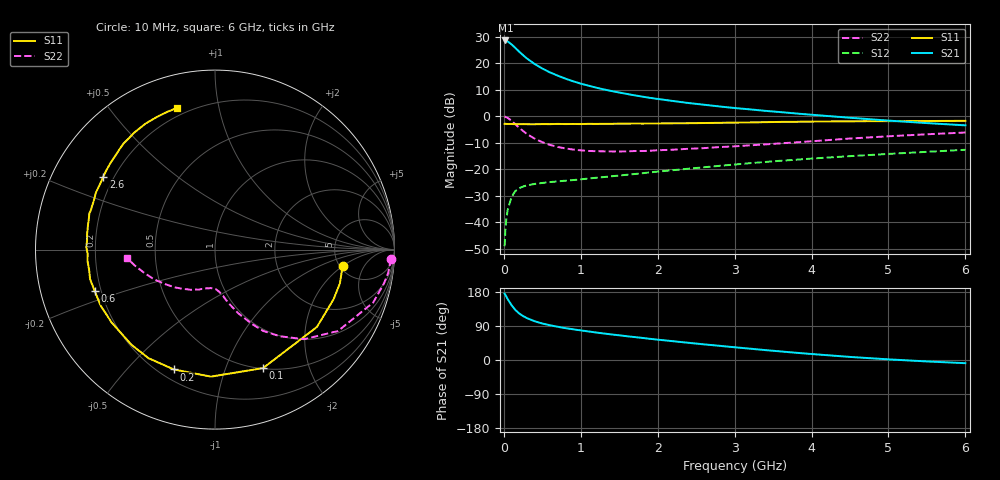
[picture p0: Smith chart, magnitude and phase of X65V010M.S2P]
! SIEMENS Small Signal Semiconductors
! BFP193W
! Si NPN RF Bipolar Junction Transistor in SOT343
! VCE = 5 V  IC = 10 mA
! Common Emitter S-Parameters:  April 1994
# GHz  S  MA  R  50
!  f  S11  S21  S12  S22
! GHz  MAG  ANG  MAG  ANG  MAG  ANG  MAG  ANG
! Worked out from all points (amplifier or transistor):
!   40 points, 10 MHz to 6 GHz, reference 50 ohm
!   highest |S21| = 28.6 dB at 20 MHz (marker M1)
!   |S21| within 3 dB of that: start of sweep to 156.1 MHz
!   unconditionally stable (mu >= 1): 1.325 GHz to 4.237 GHz
!   at 200 MHz: K = 0.22, MSG = 25.8 dB, |S12| = -27.2 dB
!   at 1.5 GHz: K = 1.05, MAG = 14.3 dB, |S12| = -22.4 dB
!   at 6 GHz: K = 0.92, MSG = 4.6 dB, |S12| = -12.7 dB
!   lowest NFmin = 1.30 dB at 450 MHz
!   S11 on the Smith chart (normalised r, x): 10 MHz: 5.28, -2.01; 100 MHz: 0.51, -1.36; 200 MHz: 0.26, -0.68; 600 MHz: 0.18, -0.16; 2.6 GHz: 0.16, +0.29; 6 GHz: 0.16, +0.76
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0.01  0.7169 -7.4  26.98 175.1  0.0035 87.1  0.9816 -3.0
0.02  0.7209 -15.2  27.01 172.0  0.0071 80.8  0.9734 -7.7
0.03  0.7163 -22.7  26.71 168.2  0.0105 80.2  0.9599 -11.4
0.05  0.7129 -37.2  25.87 160.7  0.017 73.1  0.9294 -18.5
0.1  0.7123 -67.9  22.78 144.7  0.0296 59.7  0.822 -33.5
0.15  0.7081 -91.8  19.51 131.9  0.0386 49.7  0.7036 -45.2
0.2  0.706 -108.9  16.54 122.7  0.0435 43.3  0.6029 -53.2
0.25  0.7095 -121.5  14.24 115.9  0.047 38.8  0.5264 -59.4
0.3  0.7055 -131.3  12.34 110.5  0.0492 35.7  0.4607 -63.7
0.4  0.7048 -144.8  9.714 102.3  0.0525 32.6  0.3769 -70.0
0.5  0.7098 -154.0  7.97 96.3  0.0548 31.6  0.3229 -74.3
0.6  0.7088 -161.0  6.728 91.6  0.0569 31.4  0.2869 -77.7
0.8  0.7102 -171.1  5.13 84.1  0.0605 32.8  0.2464 -82.5
1.1  0.7173 178.8  3.781 75.3  0.0665 35.8  0.2206 -88.6
1.3  0.718 173.1  3.207 69.9  0.0708 37.9  0.2167 -92.4
1.6  0.7234 166.3  2.632 62.7  0.0782 40.9  0.2169 -97.7
2.2  0.7357 154.3  1.938 49.6  0.0955 44.5  0.2329 -109.2
2.6  0.7434 146.9  1.648 41.3  0.1084 45.6  0.2493 -117.2
3.2  0.7625 136.8  1.346 29.9  0.1296 45.4  0.2817 -128.8
4.5  0.8017 118.8  0.935 8.1  0.176 41.0  0.3787 -154.1
5.5  0.8119 109.5  0.741 -3.8  0.2123 36.2  0.4559 -168.8
6  0.8171 105.0  0.672 -8.4  0.232 33.8  0.4918 -174.6
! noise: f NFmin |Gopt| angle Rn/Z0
0.45  1.3  0.22  143  0.11
0.9  1.3  0.34  160  0.11
1.8  2.05  0.54  -153  0.14
